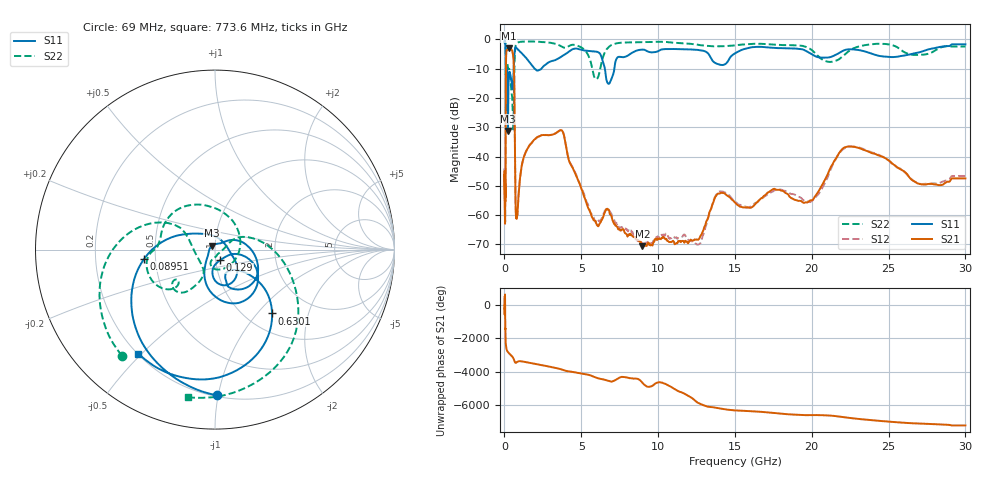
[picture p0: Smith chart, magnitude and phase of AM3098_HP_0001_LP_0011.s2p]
! Date/Time: Thu, Feb 28, 2019 8:31 AM
! Network Analyzer: Agilent Technologies E8364B Rev: A.07.50.67
! Sweep from 0.010 to 30.000 GHz, 1601 Points, Sweep Type: LOG
! Power Supply: 5.023 V, 0.002 A
# Hz S DB R 50
!freq MagS11 AngS11 MagS21 AngS21 MagS12 AngS12 MagS22 AngS22
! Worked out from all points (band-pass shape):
!   1601 points, 10 MHz to 30 GHz, reference 50 ohm
!   highest |S21| = -3.04 dB at 265.1 MHz (marker M1); lowest = -70.6 dB at 8.982 GHz (marker M2)
!   |S21| within 3 dB of the highest: 104.7 MHz to 576.6 MHz (471.9 MHz wide, 139 % of centre)
!   lowest |S11| = -31.3 dB at 227 MHz (marker M3), VSWR 1.06, Z = 48.3 + j2.11 ohm
!   |S11| at or under -10 dB: 175.3 MHz to 598.2 MHz (422.9 MHz wide, 109 % of centre); 1.975 GHz to 2.397 GHz (421.6 MHz wide, 19.3 % of centre); 6.534 GHz to 7.152 GHz (618 MHz wide, 9.03 % of centre)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
!   |S22| runs from -30.7 to -0.5 dB; largest |S21 - S12| = 0.0097
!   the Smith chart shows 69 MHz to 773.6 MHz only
!   S11 on the Smith chart (normalised r, x): 69 MHz: 0.21, -0.99; 89.51 MHz: 0.43, -0.05; 129 MHz: 1.05, -0.13; 630.1 MHz: 1.31, -1.20; 773.6 MHz: 0.20, -0.49
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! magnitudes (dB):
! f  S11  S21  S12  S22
! 10 MHz  -0.3  -46.2  -47.6  -0.5
! 38.04 MHz  -0.5  -61.5  -61.3  -0.9
! 69 MHz  -1.8  -52.2  -51.1  -2.1
! 89.51 MHz  -8.0  -18.9  -18.8  -9.5
! 98.93 MHz  -24.1  -7.8  -7.8  -17.1
! 129 MHz  -23.6  -4.0  -4.0  -11.3
! 144.7 MHz  -13.4  -3.6  -3.6  -10.2
! 186.8 MHz  -11.5  -3.5  -3.5  -8.2
! 227 MHz  -31.3  -3.1  -3.1  -9.8
! 265.1 MHz  -14.9  -3.0  -3.0  -10.2
! 550.5 MHz  -15.8  -5.0  -4.9  -27.3
! 630.1 MHz  -6.4  -12.7  -12.7  -13.1
! 717.7 MHz  -2.7  -54.4  -55.4  -2.4
! 773.6 MHz  -2.8  -60.4  -60.0  -1.6
! 2.084 GHz  -10.6  -33.6  -33.7  -0.7
! 3.723 GHz  -5.8  -31.0  -31.0  -2.4
! 5.959 GHz  -4.2  -62.8  -62.2  -13.6
! 7.926 GHz  -5.8  -66.5  -65.0  -1.0
! 8.982 GHz  -3.5  -70.6  -69.8  -0.9
! 19.61 GHz  -3.8  -55.6  -55.4  -2.5
! 22.67 GHz  -3.4  -36.7  -36.6  -3.1
! 30 GHz  -1.7  -47.5  -46.6  -2.4
